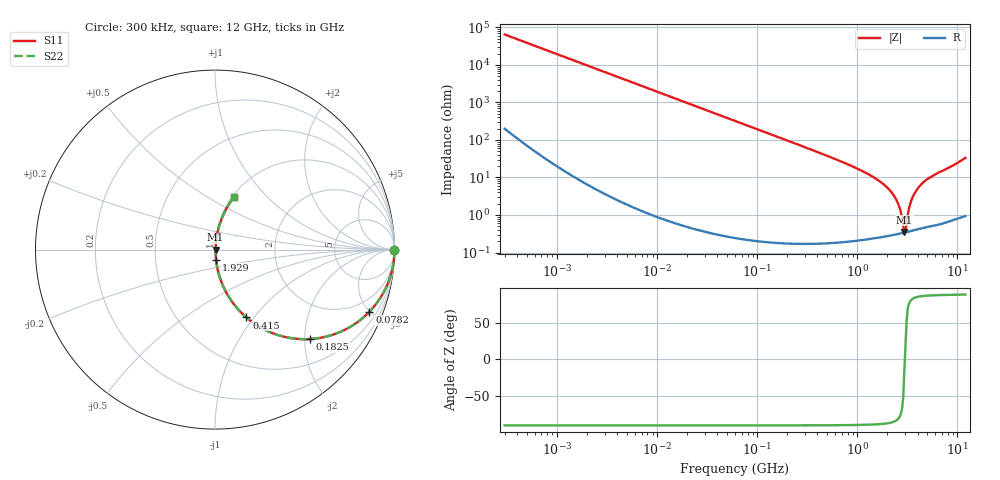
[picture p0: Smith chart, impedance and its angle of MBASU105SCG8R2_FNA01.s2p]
! MBASU105SCG8R2_FNA01  S-PARAMETER MODEL  ( Standard Model )
! Model Generated by TAIYO YUDEN Corporation (http://www.ty-top.com)
! Version 1.0
! TAIYO YUDEN Control No. 230609
! Copyright(c) 2023 TAIYO YUDEN CO.,LTD. All Rights Reserved.
! Product Description (link to TY-COMPAS)
! https://ds.yuden.co.jp/TYCOMPAS/or/detail?pn=MBASU105SCG8R2DFNA01&u=M
! Products Name : Multilayer Ceramic Capacitors
! Characteristics :
!  Capacitance : 8.2 [pF] , Rated Voltage : 50 [V] , TCC : CG / C0G
!  Case Size : 1.0 x 0.5 / 0.039 x 0.02 [mm/inch] , Thickness : 0.5 / 0.02 [mm/inch]
!  (Conditions: Temperature = 25 [degC] , DC Bias Voltage = 0 [V])
! External Node Assignments :
!  1  o---| |---o  2
! GND o---------o GND
! Frequency Range : 0.3MHz  -  12000MHz  [ 401 STEP ]
# MHZ S RI R 50
! Freq[MHz].  S11 Real  S11 Imag  S21 Real  S21 Imag  S12 Real  S12 Imag  S22 Real  S22 Imag
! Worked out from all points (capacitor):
!   401 points, 300 kHz to 12 GHz, reference 50 ohm
!   read as one part in series: C = 8.2 pF near 316.3 kHz
!   lowest |Z| = 352 mohm at 2.947 GHz (marker M1)
!   series resonance near 2.983 GHz, so ESL is about 350 pH
!   S11 on the Smith chart (normalised r, x): 300 kHz: open; 78.2 MHz: 1.00, -4.96; 182.5 MHz: 1.00, -2.12; 415 MHz: 1.00, -0.92; 1.929 GHz: 1.01, -0.12; 12 GHz: 1.02, +0.67
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0.3  1 -0.00155  7.15e-06 0.00155  7.15e-06 0.00155  1 -0.00155
1.769972  0.9999 -0.00912  8.97e-05 0.00912  8.97e-05 0.00912  0.9999 -0.00912
10.44266  0.9971 -0.0536  0.00291 0.0536  0.00291 0.0536  0.9971 -0.0536
27.10171  0.9808 -0.137  0.0192 0.137  0.0192 0.137  0.9808 -0.137
60  0.9125 -0.2821  0.0875 0.2821  0.0875 0.2821  0.9125 -0.2821
78.19928  0.86 -0.3466  0.14 0.3466  0.14 0.3466  0.86 -0.3466
182.544  0.5287 -0.4983  0.4713 0.4983  0.4713 0.4983  0.5287 -0.4983
353.9943  0.2268 -0.4172  0.7732 0.4172  0.7732 0.4172  0.2268 -0.4172
414.98  0.1747 -0.3778  0.8253 0.3778  0.8253 0.3778  0.1747 -0.3778
1105.905  0.0243 -0.1472  0.9757 0.1472  0.9757 0.1472  0.0243 -0.1472
1928.972  0.00603 -0.0576  0.994 0.0576  0.994 0.0576  0.00603 -0.0576
2088.533  0.00497 -0.0466  0.995 0.0466  0.995 0.0466  0.00497 -0.0466
2514.07  0.00355 -0.0217  0.9965 0.0217  0.9965 0.0217  0.00355 -0.0217
2650.866  0.00339 -0.0147  0.9966 0.0147  0.9966 0.0147  0.00339 -0.0147
2870.14  0.00335 -0.00439  0.9967 0.00439  0.9967 0.00439  0.00335 -0.00439
2947.191  0.00338 -0.000915  0.9966 0.000915  0.9966 0.000915  0.00338 -0.000915
3107.553  0.00352 0.00457  0.9965 -0.00457  0.9965 -0.00457  0.00352 0.00457
3364.605  0.00405 0.0189  0.996 -0.0189  0.996 -0.0189  0.00405 0.0189
3547.679  0.00463 0.0283  0.9954 -0.0283  0.9954 -0.0283  0.00463 0.0283
4270.516  0.00813 0.0613  0.9919 -0.0613  0.9919 -0.0613  0.00813 0.0613
5868.704  0.0186 0.1147  0.9814 -0.1147  0.9814 -0.1147  0.0186 0.1147
12000  0.1064 0.2946  0.8936 -0.2946  0.8936 -0.2946  0.1064 0.2946
